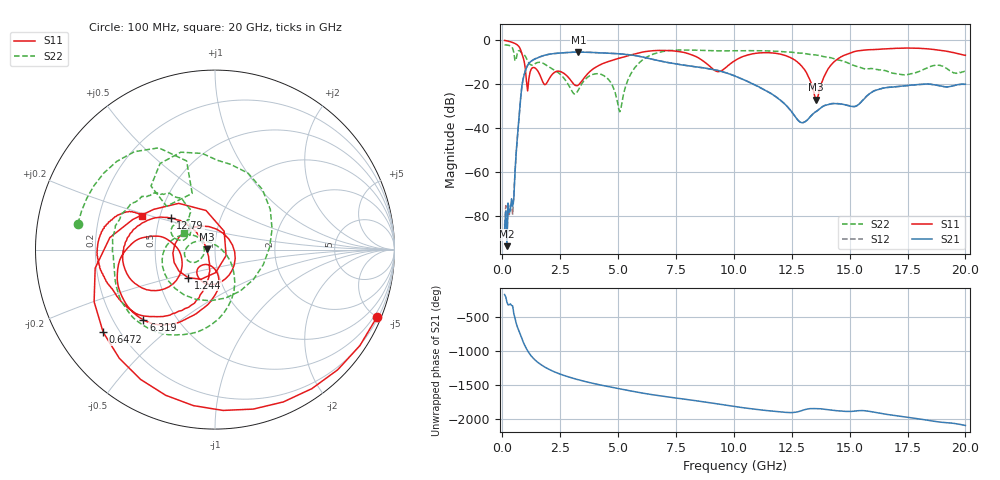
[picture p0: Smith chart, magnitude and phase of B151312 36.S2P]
!  2-Port S-parameters saved by WinCal
! VAR MeasName=S-Parameters (CALIBRATED_DATA) read from VNA (N5244A)
! VAR MeasDate=12/8/2015 5:46:27 PM
! VAR NAME=B151312 36
! VAR FILENAME=B151312 36.S2P
! VAR DATE=12/8/2015 5:46:27 PM
! VAR PHYS_PORTS=1,2
# Hz S DB R 50
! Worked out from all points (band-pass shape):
!   401 points, 100 MHz to 20 GHz, reference 50 ohm
!   highest |S21| = -5.48 dB at 3.284 GHz (marker M1); lowest = -93.5 dB at 199.5 MHz (marker M2)
!   |S21| within 3 dB of the highest: 1.432 GHz to 6.378 GHz (4.946 GHz wide, 127 % of centre)
!   lowest |S11| = -27.0 dB at 13.53 GHz (marker M3), VSWR 1.09, Z = 45.7 + j0.075 ohm
!   |S11| at or under -10 dB: 950.3 MHz to 4.517 GHz (3.567 GHz wide, 130 % of centre); 8.737 GHz to 9.948 GHz (1.21 GHz wide, 13 % of centre); 12.75 GHz to 14.32 GHz (1.568 GHz wide, 11.6 % of centre)
!   |S22| runs from -32.5 to -2.2 dB; largest |S21 - S12| = 0.0021
!   S11 on the Smith chart (normalised r, x): 100 MHz: 0.29, -4.99; 647.2 MHz: 0.14, -0.32; 1.244 GHz: 0.71, -0.23; 6.319 GHz: 0.33, -0.37; 12.79 GHz: 0.57, +0.22; 20 GHz: 0.40, +0.19
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1e8  -0.20 -22.6  -85.57 -174.5  -84.13 130.2  -2.19 169.3
1.995e8  -0.38 -44.4  -93.53 75.6  -90.31 31.5  -2.28 158.2
3.985e8  -0.94 -87.1  -72.03 25.9  -74.58 7.8  -3.01 129.5
6.4725e8  -2.22 -143.5  -44.64 74.2  -44.69 74.0  -5.98 135.2
8.96e8  -7.78 146.6  -17.82 -143.2  -17.82 -143.2  -6.32 79.7
1.24425e9  -13.29 -133.9  -9.62 7.9  -9.63 7.9  -11.33 -37.8
1.5925e9  -15.14 135.4  -7.77 -102.9  -7.77 -102.9  -10.09 -146.0
1.9905e9  -18.20 -23.8  -6.52 174.5  -6.52 174.5  -12.02 168.9
2.5875e9  -14.66 -118.2  -5.82 89.3  -5.82 89.3  -16.44 147.3
3.284e9  -20.43 -101.0  -5.48 17.4  -5.48 17.4  -22.73 -153.5
3.43325e9  -18.63 -87.5  -5.50 4.0  -5.49 4.0  -19.83 -146.8
4.3785e9  -10.52 -95.9  -5.89 -69.0  -5.88 -69.0  -16.12 175.0
5.075e9  -8.20 -108.8  -6.26 -115.9  -6.25 -115.8  -32.54 57.4
6.31875e9  -5.05 -135.6  -8.32 166.9  -8.31 166.8  -7.30 -95.2
6.7665e9  -4.72 -147.6  -9.40 144.2  -9.40 144.0  -5.60 -114.9
1.005e10  -9.29 -141.6  -16.36 -16.3  -16.33 -16.1  -4.86 -178.9
1.278625e10  -10.39 144.6  -36.54 -90.1  -36.56 -90.0  -5.93 146.0
1.338325e10  -20.99 143.7  -33.91 -44.7  -33.87 -44.6  -6.66 138.1
1.35325e10  -27.04 178.9  -32.55 -45.5  -32.59 -45.3  -6.76 136.2
1.45275e10  -8.27 -118.5  -28.92 -78.6  -28.87 -78.9  -9.12 124.6
1.67165e10  -3.93 -166.2  -21.47 -135.4  -21.38 -136.2  -14.53 136.2
2e10  -6.96 155.2  -20.07 68.0  -20.14 67.6  -14.14 151.3
